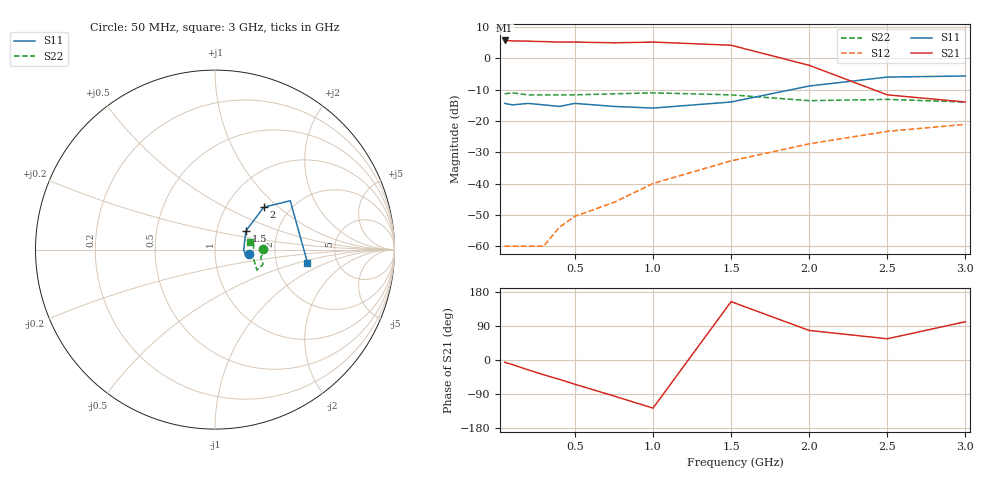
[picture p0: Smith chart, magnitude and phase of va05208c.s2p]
!  IVA-05208  S PARAMETERS
!  S PARAMETERS (VGC=4.0V, Id=32.5 mA)!  LAST UPDATED 08-11-93
# ghz s ma r 50
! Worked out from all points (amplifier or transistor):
!   12 points, 50 MHz to 3 GHz, reference 50 ohm
!   highest |S21| = 5.7 dB at 50 MHz (marker M1)
!   |S21| within 3 dB of that: start of sweep to 1.615 GHz
!   unconditionally stable (mu >= 1): start of sweep to end of sweep
!   at 200 MHz: K = 240.29, MAG = 5.9 dB, |S12| = -60.0 dB
!   at 750 MHz: K = 51.13, MAG = 5.4 dB, |S12| = -46.0 dB
!   at 3 GHz: K = 20.01, MAG = -12.5 dB, |S12| = -21.1 dB
!   S11 on the Smith chart (normalised r, x): 50 MHz: 1.46, -0.07; 1.5 GHz: 1.38, +0.30; 2 GHz: 1.48, +0.81; 3 GHz: 3.03, -0.60
0.05  0.19 -7.0  1.92 -6.0  0.001 92.0  0.27 1.0
0.1  0.18 -6.0  1.89 -12.0  0.001 54.0  0.28 -4.0
0.2  0.19 -7.0  1.87 -26.0  0.001 80.0  0.26 -8.0
0.3  0.18 -9.0  1.84 -39.0  0.001 103.0  0.26 -9.0
0.4  0.17 -10.0  1.81 -51.0  0.002 109.0  0.26 -10.0
0.5  0.19 -11.0  1.81 -64.0  0.003 110.0  0.26 -11.0
0.75  0.17 -8.0  1.76 -95.0  0.005 131.0  0.27 -14.0
1  0.16 -1.0  1.81 -127.0  0.01 137.0  0.28 -17.0
1.5  0.2 31.0  1.61 154.0  0.023 130.0  0.26 -26.0
2  0.36 41.0  0.77 78.0  0.043 113.0  0.21 -8.0
2.5  0.5 33.0  0.26 56.0  0.068 102.0  0.22 8.0
3  0.52 -8.0  0.2 101.0  0.088 72.0  0.2 12.0
